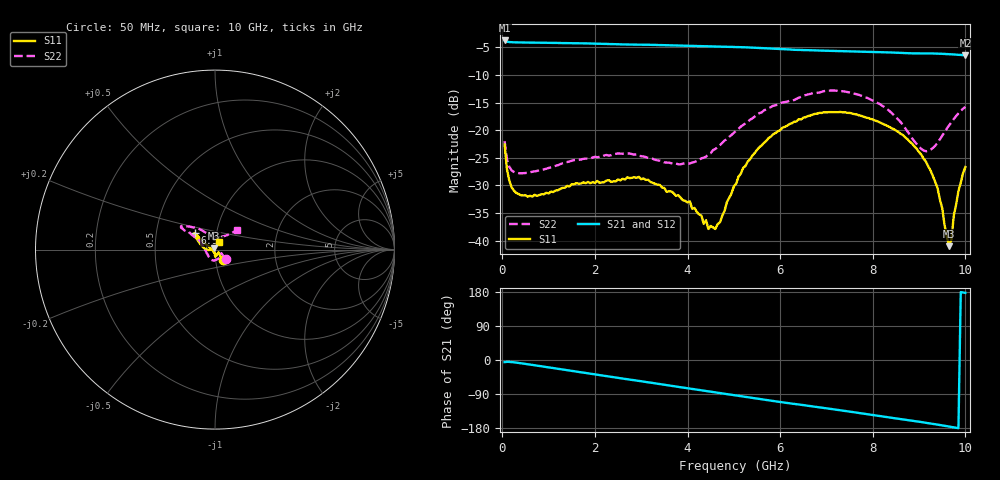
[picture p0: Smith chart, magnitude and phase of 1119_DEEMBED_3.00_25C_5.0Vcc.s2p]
!Hittite Microwave Corp.
!Digital Attenuator/PhaseShifter Rev 1.4.0
!Filename: C:\DATA\DATA\1119_DEEMBED_3.00_25C_5.0Vcc.s2p
!VNA ID: Agilent Technologies,N5224A,MY51441122,A.10.45.03
!Device type:
!2 Port Calibration.
!Temp(C): 25
!Lot Number:
!Serial Number:
!Operator:
!Misc:
!Attenuator:  3.000
# GHZ S DB R 50.0
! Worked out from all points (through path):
!   200 points, 50 MHz to 10 GHz, reference 50 ohm
!   highest |S21| = -3.73 dB at 50 MHz (marker M1); lowest = -6.4 dB at 10 GHz (marker M2)
!   group delay of S21, straight-line fit = 49.9 ps
!   lowest |S11| = -41.0 dB at 9.65 GHz (marker M3), VSWR 1.02, Z = 49.6 + j0.787 ohm
!   |S11| at or under -10 dB: start of sweep to end of sweep
!   |S22| runs from -27.8 to -12.8 dB; largest |S21 - S12| = 0.0015
!   S11 on the Smith chart (normalised r, x): 50 MHz: 1.09, -0.13; 6.95 GHz: 0.78, +0.15; 10 GHz: 1.05, +0.08
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0.05  -22.62 -52.3  -3.73 -5.7  -3.72 -5.7  -21.98 -41.5
0.15  -29.11 -46.1  -4.02 -4.9  -4.02 -4.9  -26.62 -32.7
0.4  -31.78 -37.5  -4.09 -8.5  -4.09 -8.5  -27.81 -29.4
1.75  -29.45 -81.8  -4.26 -33.4  -4.26 -33.4  -25.19 -74.2
2.95  -28.46 -88.8  -4.49 -55.2  -4.49 -55.2  -24.64 -115.5
3.4  -29.90 -90.7  -4.54 -63.5  -4.55 -63.5  -25.52 -130.6
4.05  -32.89 -92.2  -4.69 -75.4  -4.70 -75.4  -26.05 -162.2
4.45  -37.90 -124.4  -4.80 -82.7  -4.82 -82.7  -24.35 172.5
4.6  -37.91 -149.1  -4.83 -85.3  -4.85 -85.3  -23.40 163.6
5.05  -29.68 157.9  -4.92 -93.4  -4.94 -93.5  -20.11 150.3
5.75  -21.43 146.5  -5.16 -106.3  -5.18 -106.4  -15.99 147.1
6.7  -17.18 141.5  -5.51 -122.5  -5.52 -122.5  -13.32 147.1
6.95  -16.74 141.2  -5.58 -126.6  -5.59 -126.6  -12.91 146.9
7.7  -17.30 145.4  -5.75 -139.8  -5.75 -139.8  -13.59 141.4
8.35  -19.36 152.2  -5.90 -151.5  -5.90 -151.5  -16.44 128.5
8.999999  -23.96 170.7  -6.07 -162.9  -6.07 -162.9  -23.01 106.0
9.25  -27.35 -178.4  -6.09 -167.6  -6.10 -167.6  -23.52 82.5
9.400001  -30.54 -176.8  -6.11 -170.6  -6.13 -170.6  -22.25 65.6
9.65  -41.02 116.9  -6.22 -175.7  -6.23 -175.7  -19.10 48.2
9.7  -39.73 89.7  -6.25 -176.7  -6.26 -176.7  -18.53 46.4
9.85  -31.02 62.4  -6.33 -179.8  -6.34 -179.8  -16.94 43.6
10  -26.66 59.2  -6.42 177.2  -6.42 177.2  -15.77 42.0
